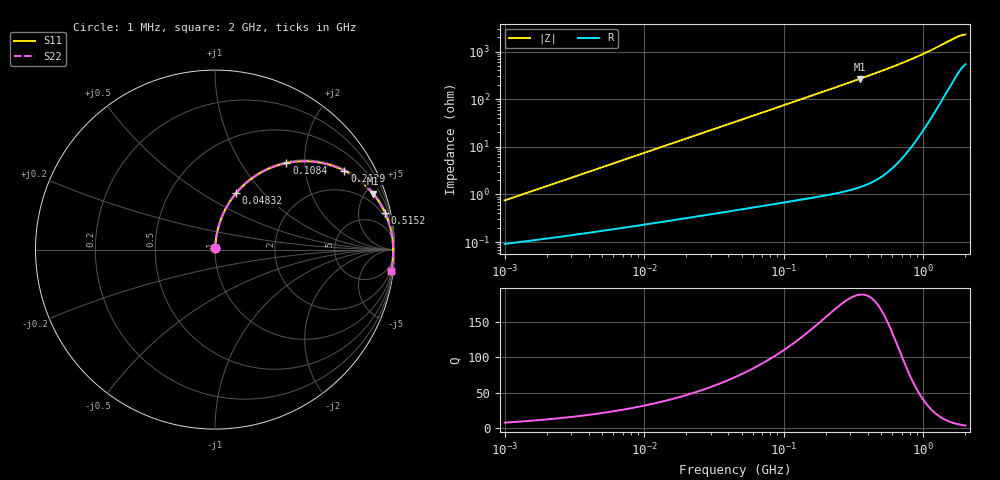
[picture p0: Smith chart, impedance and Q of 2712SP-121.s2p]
# MHz  S  MA  R  50
!Freq  MagS11  AngS11  MagS21  AngS21  MagS12  AngS12  MagS22  AngS22
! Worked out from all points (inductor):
!   801 points, 1 MHz to 2 GHz, reference 50 ohm
!   read as one part in series: L = 119 nH near 1.039 MHz
!   highest Q = 188 at 348.9 MHz (marker M1), where L = 121 nH
!   S11 on the Smith chart (normalised r, x): 1 MHz: 1.00, +0.01; 48.32 MHz: 1.01, +0.72; 108.4 MHz: 1.02, +1.62; 212.9 MHz: 1.06, +3.25; 515.2 MHz: 1.35, +9.11; 2 GHz: 2, -17
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1  0.007469 82.5  0.9991 -0.4  0.9991 -0.4  0.007469 82.5
3.573795  0.02651 85.2  0.9982 -1.5  0.9982 -1.5  0.02651 85.2
7.152559  0.05293 84.8  0.9966 -3.1  0.9966 -3.1  0.05293 84.8
12.65119  0.09326 83.0  0.9931 -5.4  0.9931 -5.4  0.09325 83.0
24.14483  0.1758 78.7  0.981 -10.2  0.981 -10.2  0.1758 78.7
33.67428  0.2416 75.0  0.9665 -14.1  0.9665 -14.1  0.2415 75.0
44.78507  0.3142 70.7  0.945 -18.5  0.945 -18.5  0.3141 70.7
48.32323  0.3362 69.4  0.9373 -19.8  0.9373 -19.8  0.3362 69.4
72.03191  0.4696 61.1  0.8778 -28.2  0.8778 -28.2  0.4696 61.1
108.3981  0.6249 50.5  0.7753 -39.0  0.7753 -39.0  0.6249 50.5
132.3446  0.6991 44.8  0.7096 -44.8  0.7096 -44.8  0.699 44.8
160.0527  0.7638 39.3  0.6401 -50.3  0.6401 -50.3  0.7637 39.3
212.8619  0.8446 31.3  0.5303 -58.3  0.5303 -58.3  0.8445 31.3
272.5345  0.8968 25.1  0.4375 -64.6  0.4375 -64.6  0.8967 25.1
348.9355  0.9339 19.5  0.3527 -70.2  0.3527 -70.2  0.9338 19.5
515.2125  0.969 12.3  0.2414 -77.4  0.2414 -77.4  0.9688 12.3
566.5845  0.9744 10.7  0.2185 -78.9  0.2185 -78.9  0.9742 10.7
813.0595  0.9875 5.6  0.145 -83.6  0.145 -83.6  0.9873 5.6
1112.605  0.9921 1.5  0.09609 -86.5  0.09609 -86.5  0.9919 1.5
1706.449  0.9909 -4.2  0.05038 -85.5  0.05038 -85.5  0.991 -4.2
1858.848  0.9897 -5.6  0.04547 -84.2  0.04547 -84.2  0.9899 -5.6
2000  0.9882 -6.8  0.04328 -83.1  0.04328 -83.1  0.9886 -6.9
